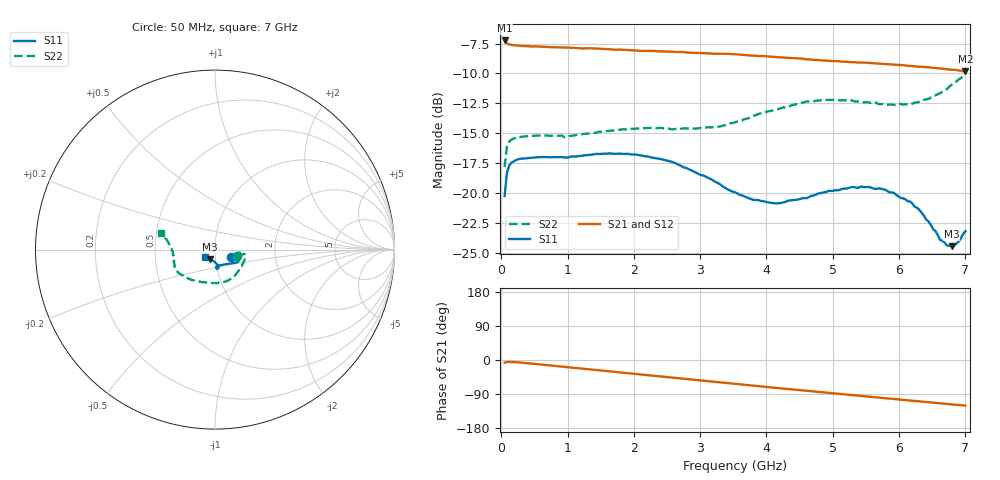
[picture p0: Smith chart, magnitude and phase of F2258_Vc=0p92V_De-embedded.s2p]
! Integrated Device Technology
! Corporate Headquarters
! 6024 Silver Creek Valley Road
! San Jose, CA 95138  USA
! Phone:  1-408-284-8200
! Toll Free:  1-800-223-1366
! Webpage:  http://www.idt.com/
! Timing and RF Division
! 515 Groton Road, Suite 102
! Westford, MA 01886-6024
! Device:  F2258
! Description: Voltage Variable RF Attenuator
! Frequency:  50.0 -  6000.00 MHz
! Package:  3x3 mm Thin QFN Plastic Package: 16 pin
! Ports:  2 RF, 2 DC
!  Pin  1  = NC
!  Pin  2  = NC
!  Pin  3  = RF2  = Port 2
!  Pin  4  = GND
!  Pin  5  = Vdd
!  Pin  6  = NC
!  Pin  7  = VCTRL
!  Pin  8  = NC
!  Pin  9  = GND
!  Pin 10  = RF1  = Port 1
!  Pin 11  = NC
!  Pin 12  = NC
!  Pin 13  = NC
!  Pin 14  = NC
!  Pin 15  = NC
!  Pin 16  = NC
! Vcntrl:  0.920 Volts
! Vdd:  +3.300 Volts
! Current:  1.148 mA
! Data:  The device was measured on a the F2258 evaluation board which has
!  individual transmission lines to the RF pins.  Data was collected
!  using a calibrated network analyzer.  The evaluation board was
!  de-embedded using a TRL calibration technique.
!  The reference plane is the edge of the package pin.
! Misc:  SN 10
!  Action Tracker AT0285
! Date Measured:  2014-12-10
! Date:  2016-01-13  MJV
! Note:
!  Integrated Device Technology supplies this data as a sample of measured
!  data at the package pin for this product.  Your particular data for this
!  product may vary.
!  Data was taken at 25 degrees C.
!  Integrated Device Technology reserves the right to change this data at anytime.
!Freq_(GHz)  S11M_(dB)  S11P_(deg)  S21M_(dB)  S21P_(deg)  S12M_(dB)  S12P_(deg)  S22M_(dB)  S22P_(deg)
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# GHz S dB R 50
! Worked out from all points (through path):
!   201 points, 50 MHz to 7 GHz, reference 50 ohm
!   highest |S21| = -7.24 dB at 50 MHz (marker M1); lowest = -9.8 dB at 7 GHz (marker M2)
!   group delay of S21, straight-line fit = 47.3 ps
!   lowest |S11| = -24.4 dB at 6.792 GHz (marker M3), VSWR 1.13, Z = 47 - j5.02 ohm
!   |S11| at or under -10 dB: start of sweep to end of sweep
!   |S22| runs from -17.8 to -10.0 dB; largest |S21 - S12| = 0.0021
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0.05  -20.25 -25.6  -7.24 -7.2  -7.26 -7.2  -17.82 -16.7
0.08475  -18.29 -12.4  -7.49 -5.5  -7.50 -5.5  -16.14 -9.6
0.1195  -17.69 -8.7  -7.57 -5.1  -7.58 -5.1  -15.68 -8.5
0.22375  -17.23 -7.0  -7.65 -5.9  -7.65 -5.9  -15.36 -9.8
0.9535  -17.02 -18.3  -7.83 -18.2  -7.80 -18.2  -15.33 -33.2
1.2315  -16.87 -21.4  -7.91 -23.0  -7.87 -23.0  -15.05 -41.8
1.89175  -16.72 -27.2  -8.03 -34.3  -8.04 -34.3  -14.68 -59.8
2.37825  -17.13 -31.0  -8.15 -42.7  -8.14 -42.7  -14.55 -73.4
2.93425  -18.28 -37.9  -8.28 -52.4  -8.25 -52.4  -14.62 -91.9
3.525  -19.93 -54.1  -8.39 -62.9  -8.40 -62.9  -14.08 -115.2
3.803  -20.57 -65.0  -8.51 -67.8  -8.49 -67.8  -13.54 -125.7
4.1505  -20.86 -76.3  -8.64 -73.8  -8.63 -73.8  -12.98 -136.1
4.7065  -20.20 -86.1  -8.86 -83.2  -8.83 -83.2  -12.33 -148.9
5.2625  -19.53 -85.3  -9.05 -92.2  -9.02 -92.3  -12.21 -157.9
5.43625  -19.43 -83.2  -9.09 -95.1  -9.08 -95.1  -12.40 -160.7
5.85325  -19.92 -79.1  -9.24 -101.8  -9.21 -101.9  -12.59 -169.3
6.166  -20.70 -79.3  -9.36 -106.9  -9.35 -106.9  -12.58 -176.5
6.444  -22.36 -86.1  -9.47 -111.5  -9.48 -111.5  -12.13 176.2
6.61775  -23.91 -96.7  -9.57 -114.2  -9.56 -114.3  -11.64 171.5
6.7915  -24.43 -117.7  -9.69 -117.0  -9.67 -117.1  -10.95 167.4
6.89575  -24.07 -132.1  -9.74 -118.7  -9.73 -118.7  -10.50 165.4
7  -23.18 -145.5  -9.82 -120.2  -9.80 -120.3  -10.03 163.4
